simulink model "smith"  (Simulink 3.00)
settings: Solver=ode45  StartTime=0.0  StopTime=40  RelTol=1e-6

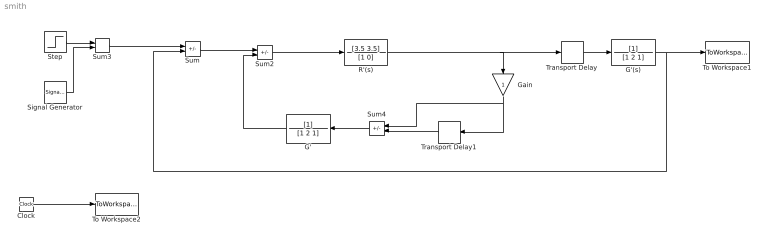
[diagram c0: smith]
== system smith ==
  Clock : Clock
  G' : TransferFcn  Orientation=left  Numerator=[1]  Denominator=[1 2 1]
  G'(s) : TransferFcn  Numerator=[1]  Denominator=[1 2 1]
  Gain : Gain  Orientation=down  Gain=1  SaturateOnIntegerOverflow=on
  R'(s) : TransferFcn  Numerator=[3.5 3.5]  Denominator=[1 0]
  Signal Generator : SignalGenerator  WaveForm=sine  Amplitude=0  Frequency=1  Units=Hertz
  Step : Step  Time=0  Before=0  After=1  SampleTime=0
  Sum : Sum  Inputs=+-  SaturateOnIntegerOverflow=on
  Sum2 : Sum  Inputs=+-  SaturateOnIntegerOverflow=on
  Sum3 : Sum  Inputs=++  SaturateOnIntegerOverflow=on
  Sum4 : Sum  Orientation=left  Inputs=+-  SaturateOnIntegerOverflow=on
  To Workspace1 : ToWorkspace  VariableName=y  SampleTime=-1  SaveFormat=Matrix
  To Workspace2 : ToWorkspace  VariableName=t  SampleTime=-1  SaveFormat=Matrix
  Transport Delay : TransportDelay  DelayTime=4  InitialInput=0  BufferSize=1024
  Transport Delay1 : TransportDelay  Orientation=left  DelayTime=4  InitialInput=0  BufferSize=1024
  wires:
  Sum2/1 -> R'(s)/1
  G'(s)/1 -> To Workspace1/1, Sum/2
  Transport Delay/1 -> G'(s)/1
  Clock/1 -> To Workspace2/1
  Step/1 -> Sum3/1
  Signal Generator/1 -> Sum3/2
  Sum3/1 -> Sum/1
  Sum/1 -> Sum2/1
  G'/1 -> Sum2/2
  Transport Delay1/1 -> Sum4/2
  Sum4/1 -> G'/1
  R'(s)/1 -> Transport Delay/1, Gain/1
  Gain/1 -> Sum4/1, Transport Delay1/1
